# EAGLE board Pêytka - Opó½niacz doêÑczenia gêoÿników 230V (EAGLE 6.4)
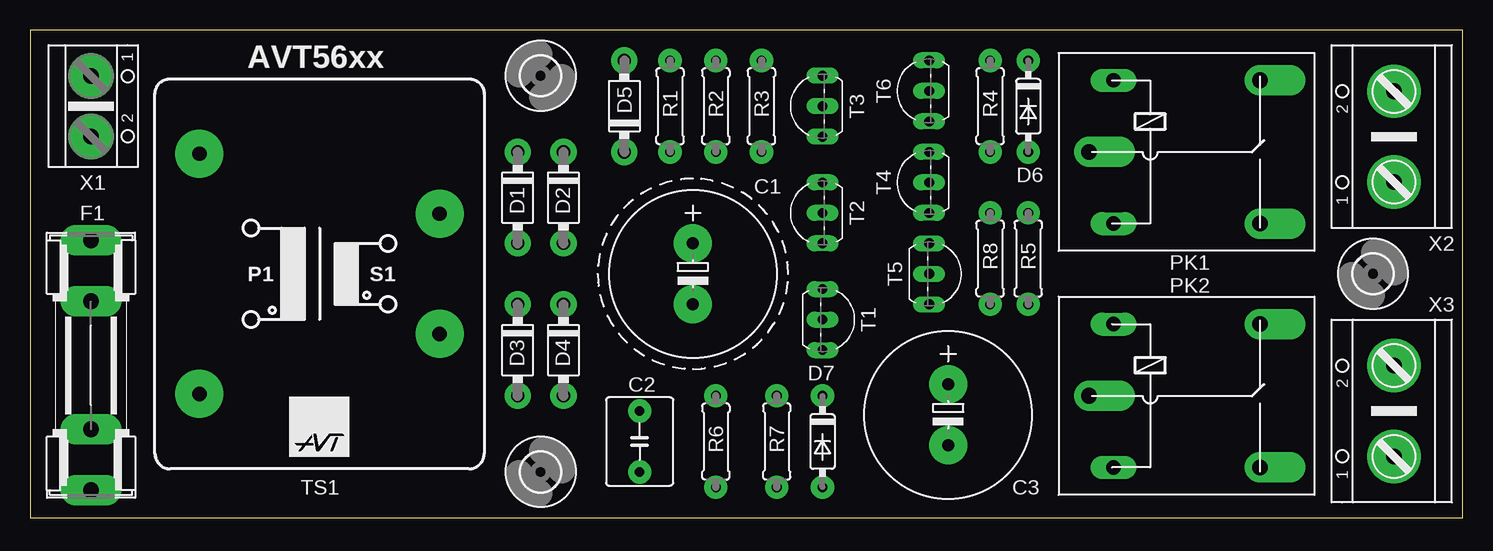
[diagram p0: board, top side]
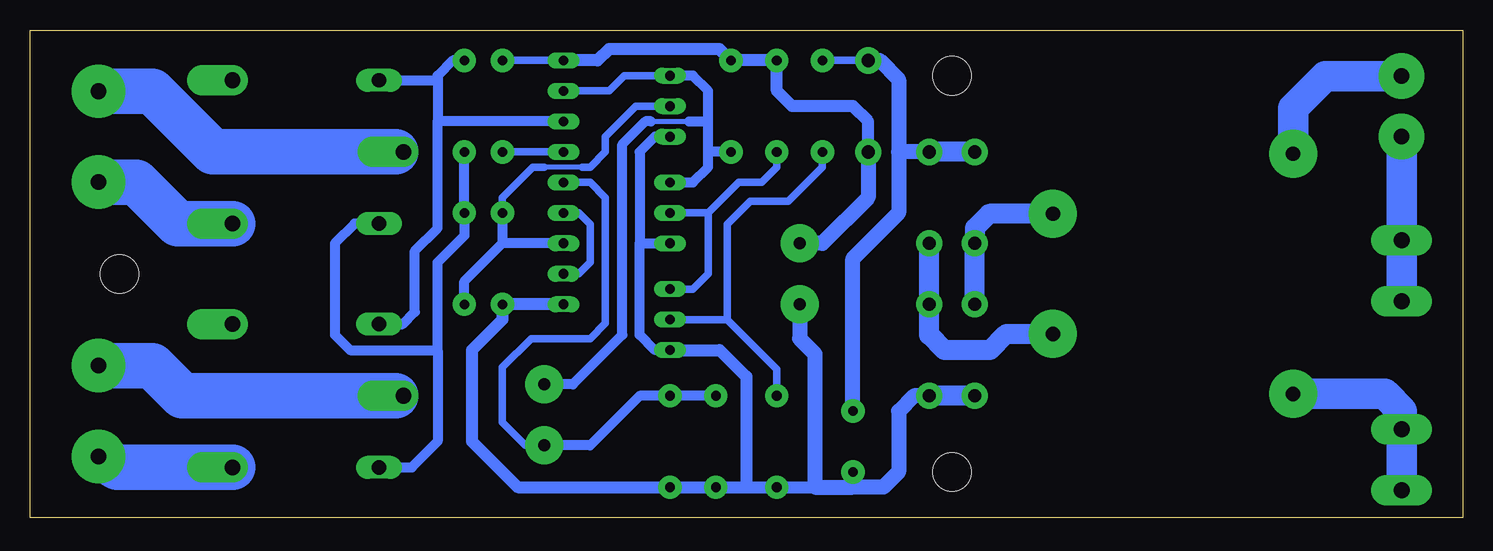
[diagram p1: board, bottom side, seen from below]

Size 119.38 x 40.64 mm. Coordinates in mm from the lower left corner, seen from the top.
Outline: 0,0 119.38,0 119.38,40.64 0,40.64 0,0
Copper layers (1*16): Top 0.035mm / dielectric 1.5mm / Bottom 0.035mm
Design rules "AVT": minimum track width 16mil, minimum drill 19mil, track to track 10mil, track to pad 10mil, pad to pad 10mil, via to via 10mil, smd to smd 10mil, copper to edge 20mil, drill to drill 10mil, minimum pad ring 10mil, minimum via ring 10mil, stop-mask expansion 4mil, vias tented up to drill 0mil, thermal gap 10mil

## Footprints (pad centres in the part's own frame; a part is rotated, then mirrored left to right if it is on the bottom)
E5-13 = drill 1 pad 3.175: + -2.54,0; - 2.54,0
C050-055X075 = drill 0.8 pad 1.93: 1 -2.54,0; 2 2.54,0
DO41-7.6 = drill 1.1 pad 2.184: A 3.81,0; C -3.81,0
DO35-7 = drill 0.8 pad 1.93: A 3.81,0; C -3.81,0
SHK20L = drill 1.321 pad 2.54 long: 1A -10.414,0; 1B -5.334,0; 2A 10.414,0; 2B 5.334,0
3,2_SMALL = hole 3.2: 0,0
G5LE = drill 1.2 pad 1.93 long: 1 -7.493,-5.969; 2 -7.493,5.969 | drill 1.3 pad 2.54 offset: O 4.699,5.969; P -9.525,0; S 4.699,-5.969
0207/7 = drill 0.8 pad 1.93: 1 -3.81,0; 2 3.81,0
TO92-EBC = drill 0.813 long: B 0,-1.27; C -2.54,-1.27; E 2.54,-1.27
TO92-EBC' = drill 0.813 long: B 0,-1.27; C 2.54,-1.27; E -2.54,-1.27
EI30_AVT = drill 1.2 pad 4: 1 -10.008,10.008; 5 -10.008,-10.008; 7 10.008,-5.004; 9 10.008,5.004
AK500/2 = drill 1.3 pad 3.81: 1 -2.515,0; 2 2.515,0
X2.2 = drill 1.3 pad 4.445: 1 -3.785,0; 2 3.785,0

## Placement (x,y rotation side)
C1  [E5-13]  55.24,20.32 270 top
C2  [C050-055X075]  50.8,6.35 270 top
C3  [E5-13]  76.52,8.57 270 top
D1  1N40047.62  [DO41-7.6]  40.64,26.67 270 top
D2  1N40047.62  [DO41-7.6]  44.45,26.67 270 top
D3  1N40047.62  [DO41-7.6]  40.64,13.97 270 top
D4  1N40047.62  [DO41-7.6]  44.45,13.97 270 top
D5  1N40047.62  [DO41-7.6]  49.53,34.29 90 top
D6  1N4148DO35-7  [DO35-7]  83.19,34.29 270 top
D7  1N4148DO35-7  [DO35-7]  66.04,6.35 270 top
F1  [SHK20L]  5.08,12.7 90 top
H1  MOUNT-HOLE3,2_SMALL  [3,2_SMALL]  42.55,3.81 0 top
H2  MOUNT-HOLE3,2_SMALL  [3,2_SMALL]  42.55,36.83 90 top
H3  MOUNT-HOLE3,2_SMALL  [3,2_SMALL]  111.92,20.32 0 top
PK1  G5L  [G5LE]  97.79,30.48 0 top
PK2  G5L  [G5LE]  97.79,10.16 0 top
R1  [0207/7]  53.34,34.29 90 top
R2  [0207/7]  57.15,34.29 90 top
R3  [0207/7]  60.96,34.29 90 top
R4  [0207/7]  80.01,34.29 90 top
R5  [0207/7]  83.19,21.59 90 top
R6  [0207/7]  57.15,6.35 90 top
R7  [0207/7]  62.23,6.35 90 top
R8  [0207/7]  80.01,21.59 90 top
T1  BC548A  [TO92-EBC]  67.31,16.51 270 top
T2  [TO92-EBC']  64.77,25.4 90 top
T3  [TO92-EBC']  64.77,34.29 90 top
T4  [TO92-EBC']  73.66,27.94 90 top
T5  BC548A  [TO92-EBC]  76.2,20.32 270 top
T6  [TO92-EBC']  73.66,35.56 90 top
TS1  EI30_AVT  [EI30_AVT]  24.13,20.32 0 top
U$1  LOGOSMALL  [SIZE_S]  21.59,5.08 0 top
X1  [AK500/2]  5.08,34.29 270 top
X2  ARK7.5/2  [X2.2]  113.67,31.75 90 top
X3  ARK7.5/2  [X2.2]  113.67,8.89 90 top

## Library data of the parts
C1-C3 R1-R8 = rcl
D1-D7 = diode
F1 = fuse; OC_FARNELL: unknown; OC_NEWARK: unknown
H1-H3 = holes
PK1 PK2 = relay; OC_FARNELL: unknown; OC_NEWARK: unknown
T1 T5 = transistor-npn
T2-T4 T6 = transistor
TS1 = trafo
U$1 = AVT_Logo
X1 = con-ptr500; OC_FARNELL: unknown; OC_NEWARK: unknown
X2 X3 = con-ptr750

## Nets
N$1: R1.1 R6.2 T1.B
N$2: F1.1A F1.1B TS1.5
N$4: R2.1 T1.C T2.B
N$5: D6.C PK1.2 PK2.2 T6.E
N$6: D6.A PK1.1 PK2.1 R5.2
N$7: PK1.S X2.1
N$8: C3.- D7.C R7.2 T4.B
N$9: C3.+ R3.1 T2.C T3.C T6.B
N$10: C1.+ D5.C R2.2 R3.2 R4.2 T6.C
N$11: PK1.P X2.2
N$12: PK2.S X3.1
N$13: C2.1 D1.C D2.C D5.A R1.2
N$14: PK2.P X3.2
N$15: T4.E T5.B
N$16: TS1.1 X1.1
N$17: R5.1 R8.2 T3.B T5.C
N$18: C1.- C2.2 D3.A D4.A D7.A R6.1 R7.1 R8.1 T1.E T2.E T3.E T5.E
N$19: R4.1 T4.C
N$20: F1.2A F1.2B X1.2
N$24: D1.A D3.C TS1.9
N$25: D2.A D4.C TS1.7

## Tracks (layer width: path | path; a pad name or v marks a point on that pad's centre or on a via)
N$1
  Bottom 0.61: T1.B 61.28,16.51 | 61.28,16.51 57.15,12.38 R6.2 | 61.28,16.51 61.28,24.45 59.37,26.35 56.2,26.35 53.34,29.21 R1.1
N$2
  Bottom 2.54: F1.1A F1.1B 5.08,8.89 6.5,10.31 TS1.5
N$4
  Bottom 0.61: T2.B 62.87,25.4 | 62.87,25.4 62.87,20.32 64.14,19.05 T1.C | 62.87,25.4 60.33,27.94 58.42,27.94 57.15,29.21 R2.1
N$5
  Bottom 0.813: PK2.2 88.33,16.13 87.31,17.14 87.31,22.23 85.41,24.13 85.41,33.02 | T6.E 85.41,33.02 | PK1.2 85.41,36.45 | 85.41,36.45 85.41,33.02 | D6.C 84.14,38.1 85.41,36.83 85.41,36.45
N$6
  Bottom 0.813: D6.A R5.2 83.19,23.5 85.41,21.27 85.41,13.97 | 85.41,13.97 85.41,6.35 87.57,4.19 PK2.1 | PK1.1 92.33,24.51 93.98,22.86 93.98,15.24 92.71,13.97 85.41,13.97
N$7
  Bottom 3.81: PK1.S 107.06,24.51 110.52,27.96 X2.1
N$8
  Bottom 0.61: T4.B 72.71,27.94 71.44,26.67 71.44,16.19 72.71,14.92 77.63,14.92 80.01,12.54 80.01,7.94 78.11,6.03 C3.-
  Bottom 0.813: R7.2 D7.C 68.58,10.16 72.71,6.03 C3.-
N$9
  Bottom 0.406: 67.63,33.02 64.45,33.02
  Bottom 0.61: T6.B 71.12,35.56 69.85,36.83 T3.C
  Bottom 0.813: T2.C 64.14,27.94 62.87,29.21 62.87,30.48 | 62.87,30.48 62.87,33.02 | 62.87,33.02 62.87,35.56 64.14,36.83 T3.C | C3.+ 74.14,11.11 70.01,15.24 70.01,31.11 68.1,33.02 67.63,33.02 | R3.1 62.87,30.48 | 64.45,33.02 62.87,33.02
N$10
  Bottom 0.61: T6.C R4.2
  Bottom 1.016: D5.C 49.53,33.02 50.8,34.29 55.88,34.29 57.15,35.56 R2.2 R3.2 61.91,39.05 71.12,39.05 72.07,38.1 T6.C
  Bottom 1.27: D5.C 49.53,26.67 53.34,22.86 C1.+
N$11
  Bottom 2.54: PK1.P 88.9,30.48
  Bottom 3.81: X2.2 109.19,35.53 104.14,30.48 88.9,30.48
N$12
  Bottom 3.81: X3.1 112.12,4.19 PK2.S
N$13
  Bottom 0.61: R1.2 D5.A
  Bottom 1.27: D5.A 48.58,38.1 46.99,36.51 46.99,30.48 | 46.99,30.48 46.99,25.4 50.8,21.59 C2.1 | D2.C 46.99,30.48
  Bottom 1.676: D1.C D2.C
N$14
  Bottom 2.54: PK2.P 88.9,10.16
  Bottom 3.81: X3.2 109.19,12.68 106.68,10.16 88.9,10.16
N$15
  Bottom 0.61: T5.B 73.66,20.32 72.71,21.27 72.71,24.45 73.66,25.4 T4.E
N$16
  Bottom 2.54: X1.1 11.46,36.8 14.12,34.14 TS1.1
N$17
  Bottom 0.406: 73.34,29.21 76.52,29.21
  Bottom 0.61: T3.B 68.9,34.29 71.44,31.75 71.44,30.48 72.71,29.21 73.34,29.21 | R8.2 80.01,26.67 77.47,29.21 76.52,29.21
  Bottom 0.813: T5.C 80.01,22.86 | R5.1 83.19,19.68 80.01,22.86 | R8.2 80.01,22.86
N$18
  Bottom 0.813: T1.E 67.31,13.97 68.58,15.24 68.58,22.86 | 68.58,22.86 T2.E | T3.E 67.31,31.75 68.58,30.48 68.58,22.86
  Bottom 1.016: 59.69,2.54 R7.1 D7.A 78.74,2.54 82.55,6.35 82.55,13.97 80.01,16.51 R8.1 T5.E | 59.69,2.54 R6.1 53.98,2.54 | T1.E 61.91,13.97 59.69,11.75 59.69,2.54
  Bottom 1.27: 50.8,2.54 53.98,2.54 53.98,13.65 55.24,14.92 C1.- | D4.A 45.72,10.16 46.99,8.89 46.99,3.81 48.26,2.54 50.8,2.54 | 50.8,2.54 C2.2
  Bottom 1.676: D3.A D4.A
N$19
  Bottom 0.61: T4.C R4.1
N$20
  Bottom 2.54: X1.2 F1.2A F1.2B
N$24
  Bottom 1.676: D3.C D1.A 40.64,24.13 39.45,25.32 TS1.9
N$25
  Bottom 1.016: 38.1,15.24 38.02,15.32
  Bottom 1.676: 38.1,15.24 39.37,13.97 43.18,13.97 44.45,15.24 D4.C D2.A | 38.02,15.32 TS1.7

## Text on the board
tPlace: AVT56xx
